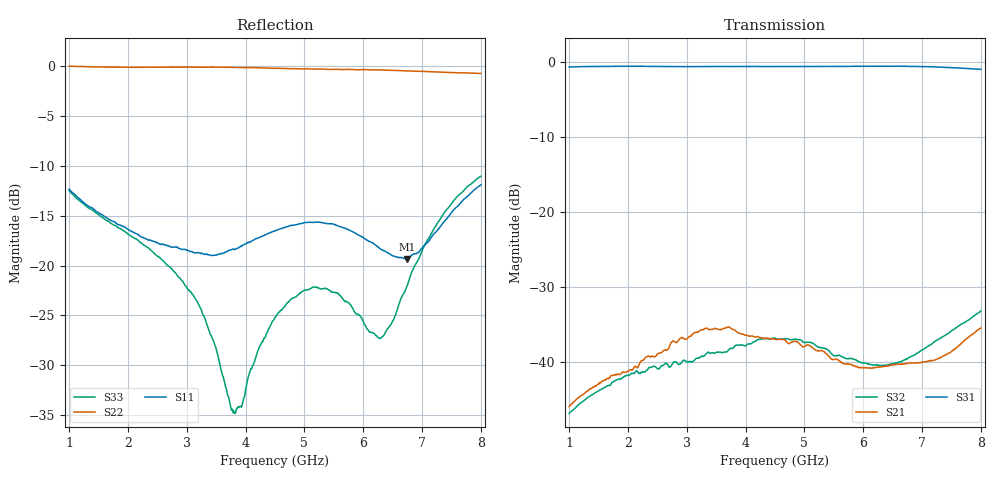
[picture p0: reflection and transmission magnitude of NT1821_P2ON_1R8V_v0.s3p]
! NT1821 PC-P2 ON state
! Port1:PC, Port2:P1, Port3:P2
! VDD=1.8V, VCTL=0V
# hz S ma R 50
! 3 Port Network Data from SP1.SP block
! freq  magS11  angS11  magS12  angS12  magS13  angS13
!  magS21  angS21
!  magS22  angS22  magS23  angS23
!  magS31  angS31  magS32  angS32
!  magS33  angS33
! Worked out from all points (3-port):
!   701 points, 1 GHz to 8 GHz, reference 50 ohm
!   strongest paths, dB at 1 GHz, 2.75 GHz, 4.5 GHz, 6.25 GHz, 8 GHz:
!     S31: -0.7, -0.6, -0.6, -0.6, -1.0
!     S21: -46.0, -37.4, -37.0, -40.7, -35.5
!     S32: -46.9, -40.4, -36.9, -40.5, -33.2
!   lowest |S11| = -19.3 dB at 6.74 GHz (marker M1), VSWR 1.24, Z = 45.1 - j9.08 ohm
!   |S11| at or under -10 dB: start of sweep to end of sweep
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1e9  0.2421 -77.8  0.005023 75.3  0.9277 1.9
     0.005012 75.3  1.002 -13.7  0.004503 72.5
     0.9272 1.7  0.004517 72.6  0.238 -76.1
1.95e9  0.1558 -82.9  0.008547 71.5  0.9395 -13.1
        0.008476 71.5  0.9896 -26.0  0.008007 64.4
        0.9381 -13.1  0.008033 64.1  0.1479 -85.6
3.1e9  0.1169 -61.3  0.01529 68.5  0.9323 -25.7
       0.01524 68.4  0.9907 -39.2  0.01003 62.8
       0.9325 -25.9  0.009984 62.7  0.0716 -94.0
3.8e9  0.1208 -38.8  0.01638 49.1  0.9342 -32.6
       0.01636 49.1  0.9869 -47.3  0.01246 63.8
       0.9345 -32.9  0.01245 63.6  0.01859 -161.9
4.5e9  0.1494 -31.1  0.01415 46.7  0.9345 -39.7
       0.0141 46.8  0.9777 -57.0  0.01429 53.1
       0.9339 -40.1  0.01434 52.8  0.05477 111.5
5.36e9  0.1628 -39.2  0.0114 43.2  0.9351 -48.3
        0.0114 43.7  0.9667 -72.7  0.01216 45.7
        0.9353 -48.6  0.01219 44.9  0.07706 100.2
6.29e9  0.1214 -74.4  0.009257 70.6  0.9391 -58.1
        0.009206 70.5  0.9583 -93.2  0.009429 69.0
        0.939 -58.5  0.009426 68.2  0.04299 155.5
6.74e9  0.108 -113.0  0.0098 82.3  0.9378 -63.2
        0.00973 82.5  0.9481 -103.0  0.01043 87.6
        0.9378 -63.9  0.01037 86.9  0.07854 -151.4
7.37e9  0.1657 -165.8  0.011 104.1  0.9231 -70.8
        0.01095 103.9  0.9344 -114.0  0.01483 103.5
        0.9232 -71.3  0.01482 103.6  0.1827 -134.7
8e9  0.2545 171.7  0.01682 118.1  0.8949 -77.9
     0.01678 117.9  0.9213 -121.8  0.02175 111.7
     0.8949 -78.4  0.02183 111.4  0.2806 -132.5
